FUNCTION_BLOCK Example35_Sectors //2x1 flyways 1 xbot (actual physical, left flyway set as master, right flyway set as sector 1) - PMC_Sector_Activate, PMC_Sector_Deactivate, PMC_Sector_Recover, PMC_Sector_GetStatus
VAR_INPUT
	Execute : BOOL;
	UserReconnectFinished : BOOL;
END_VAR
VAR_OUTPUT
	UserCanDisconnectFlyway : BOOL;
	Done : BOOL;
END_VAR
VAR_IN_OUT
	PM_Controller : PMControllerType;
END_VAR
VAR
	PMC_XYMotion1 : PMC_XYMotion;
	PMC_Sector_Deactivate1 : PMC_Sector_Deactivate;
	PMC_Sector_GetStatus1 : PMC_Sector_GetStatus; 
	PMC_XYMotion2 : PMC_XYMotion;
	PMC_Sector_Activate1 : PMC_Sector_Activate;
	PMC_Sector_Recover1 : PMC_Sector_Recover;
END_VAR

//2x1 flyways 1 xbot (actual physical, left flyway set as master, right flyway set as sector 1) - PMC_Sector_Activate, PMC_Sector_Deactivate, PMC_Sector_Recover, PMC_Sector_GetStatus

IF NOT(Execute) THEN
	UserReconnectFinished := FALSE;
END_IF; 

//move xbot 1 to the non sector flyway
PMC_XYMotion1(Execute := Execute,cmdLB := 0,XbotID := 1,Mode := 0,Type_ := 0,PosX := 0.12,PosY := 0.12,EndVel := 0,MaxVel := 1.0,MaxAcc := 10.0,PM_Controller := PM_Controller);

//deactivate sector 1
PMC_Sector_Deactivate1(Execute := PMC_XYMotion1.Done,SectorID := 1,PM_Controller := PM_Controller);
//tell user that they can disconnect the sector flyway
UserCanDisconnectFlyway := PMC_Sector_Deactivate1.Done;

//get the status of sector 1
PMC_Sector_GetStatus1(Execute := PMC_Sector_Deactivate1.Done,SectorID := 1,PM_Controller := PM_Controller);

//try to move xbot 1 to the sector flyway
PMC_XYMotion2(Execute := PMC_Sector_GetStatus1.Done,cmdLB := 0,XbotID := 1,Mode := 0,Type_ := 0,PosX := 0.36,PosY := 0.12,EndVel := 0,MaxVel := 1.0,MaxAcc := 10.0,PM_Controller := PM_Controller);

//activate sector once user says that they are done reconnecting the flyway
PMC_Sector_Activate1(Execute := UserReconnectFinished AND PMC_XYMotion2.Ack,SectorID := 1,PM_Controller := PM_Controller);

//recover sector once the sector is done activating
PMC_Sector_Recover1(Execute := PMC_Sector_Activate1.Done,SectorID := 1,PM_Controller := PM_Controller);

//Done once the xbot reaches the sector flyway
Done := PMC_XYMotion2.Done;

END_FUNCTION_BLOCK
